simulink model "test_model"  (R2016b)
settings: Solver=VariableStepAuto  StartTime=0.0  StopTime=runtime  RelTol=1e-3
InitFcn:
  | clear mex
  | delete test_model_sfun.mexw64
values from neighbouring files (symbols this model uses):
  g = 9.81    [modelParameters.m]    (also in analyzeIMU_data.m = 9.8; getMomentOfInertia.m = 9.80665)
  height_controlled_o = (((Rm*If +      + (((omega0_o * 2 * Rm * Kv * Kq       * Kd + 1)^2) - 1)/(4* Rm*Kv^2*Kq      *Kd))/Vb)*(Pmax- Pmin)+Pmin)    [modelParameters.m]
  If = 0.511    [modelParameters.m]    (also in thrustDragConstantCalculations.m = [If0; If1; If2; If3]; Kd_error.m = I_0 * sign(rotor_speed_0) + I_1 * rotor_speed_0 + I_2 * roto)
  Jreq = 4.2012e-05    [modelParameters.m]
  Jxx = 0.0130    (= 0.013)    [modelParameters.m]
  Jyy = 0.0140    (= 0.014)    [modelParameters.m]
  Jzz = 0.0285    [modelParameters.m]
  Kd = 1.0317e-7    (= 1.0317e-07)    [modelParameters.m]    (also in calcDragConstant.m = ((A'*A)^-1)*A'*b; thrustDragConstantCalculations.m = calcDragConstant(data, Pmin, Pmax, Rm, Kv, Kq, If); Kd_error.m)
  Kq = 96.3422    [modelParameters.m]    (also in thrustDragConstantCalculations.m; Kd_error.m)
  Kt = 8.6519e-6    (= 8.6519e-06)    [modelParameters.m]    (also in calcThrustConstant.m = ((A'*A)^(-1))*(A'*T); thrustDragConstantCalculations.m = calcThrustConstant(data))
  Kv = 96.3422    [modelParameters.m]    (also in thrustDragConstantCalculations.m; Kd_error.m)
  m = 1.244    [modelParameters.m]
  omega0_o = (-1 + sqrt(1 - 4*Rm*Kv*Kq*Kd*( Kv*Rm*If - Kv*Vb_eff_0))) / (2*Rm*Kv*Kq*Kd)    [modelParameters.m]
  omega1_o = (-1 + sqrt(1 - 4*Rm*Kv*Kq*Kd*( Kv*Rm*If - Kv*Vb_eff_1))) / (2*Rm*Kv*Kq*Kd)    [modelParameters.m]
  omega2_o = (-1 + sqrt(1 - 4*Rm*Kv*Kq*Kd*( Kv*Rm*If - Kv*Vb_eff_2))) / (2*Rm*Kv*Kq*Kd)    [modelParameters.m]
  omega3_o = (-1 + sqrt(1 - 4*Rm*Kv*Kq*Kd*( Kv*Rm*If - Kv*Vb_eff_3))) / (2*Rm*Kv*Kq*Kd)    [modelParameters.m]
  pitch_o = pitch_value(1)    [modelParameters.m]
  pitchrate_o = pitchrate_value(1)    [modelParameters.m]
  Pmax = 2e5    (= 200000)    [modelParameters.m]    (also in thrustDragConstantCalculations.m; Kd_error.m)
  Pmin = 1e5    (= 100000)    [modelParameters.m]    (also in thrustDragConstantCalculations.m; Kd_error.m)
  rhx = 0.16    [modelParameters.m]
  rhy = 0.16    [modelParameters.m]
  rhz = 0.03    [modelParameters.m]
  Rm = 0.2308    [modelParameters.m]    (also in thrustDragConstantCalculations.m; Kd_error.m)
  roll_o = roll_value(1)    [modelParameters.m]
  rollrate_o = rollrate_value(1)    [modelParameters.m]
  Tc = 0.04    [modelParameters.m]
  Tq = 0.005    [modelParameters.m]
  Vb = 11.1    [modelParameters.m]    (also in calcDragConstant.m = [data.(6); data.(6); data.(6); data.(6)]; Kd_error.m = data.(6))
  x_controlled_o = 0    [modelParameters.m]
  x_o = x_position(1)    [modelParameters.m]
  x_vel_o = (x_position(2) - x_position(1)) / (time(2) - time(1))    [modelParameters.m]
  y_controlled_o = 0    [modelParameters.m]
  y_o = y_position(1)    [modelParameters.m]
  y_vel_o = (y_position(2) - y_position(1)) / (time(2) - time(1))    [modelParameters.m]
  yaw_controlled_o = 0    [modelParameters.m]
  yaw_o = yaw_value(1)    [modelParameters.m]
  yawrate_o = yawrate_value(1)    [modelParameters.m]
  z_o = z_position(1)    [modelParameters.m]
  z_vel_o = (z_position(2) - z_position(1)) / (time(2) - time(1))    [modelParameters.m]
undefined symbols (not defined in the file or in its folder): DiscIntNeverNeededParam
libraries: simulink x13, vrlib x2
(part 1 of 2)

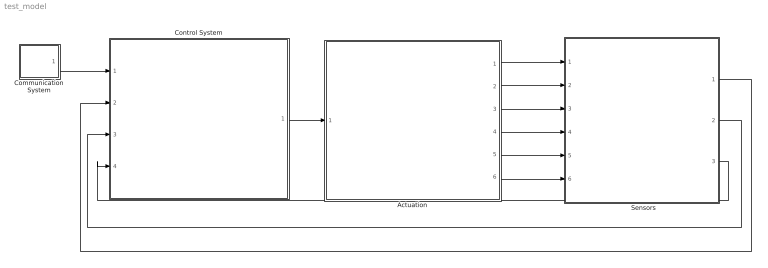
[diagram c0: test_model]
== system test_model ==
  "     Sensors   " : Subsystem
  Actuation : Subsystem
  Communication System : Subsystem
  Control System : Subsystem
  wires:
  Control System/1(P) -> Actuation/1(P)
  Communication System/1(setpoints) -> Control System/1(setpoints)
  Actuation/1(B_omega) -> "     Sensors   "/1(B_Omega)
  Actuation/2(euler_angles) -> "     Sensors   "/2(euler_angles)
  Actuation/3(B_vo) -> "     Sensors   "/3(B_vo)
  Actuation/4(E_ro) -> "     Sensors   "/4(E_ro)
  Actuation/5(B_vo_dot) -> "     Sensors   "/5(B_vo_dot)
  Actuation/6(B_g) -> "     Sensors   "/6(B_g)
  "     Sensors   "/3(current_position) -> Control System/4(current_position)
  "     Sensors   "/2(euler_rates) -> Control System/3(euler_rates)
  "     Sensors   "/1(euler_angles_filtered) -> Control System/2(euler_angles_filtered)

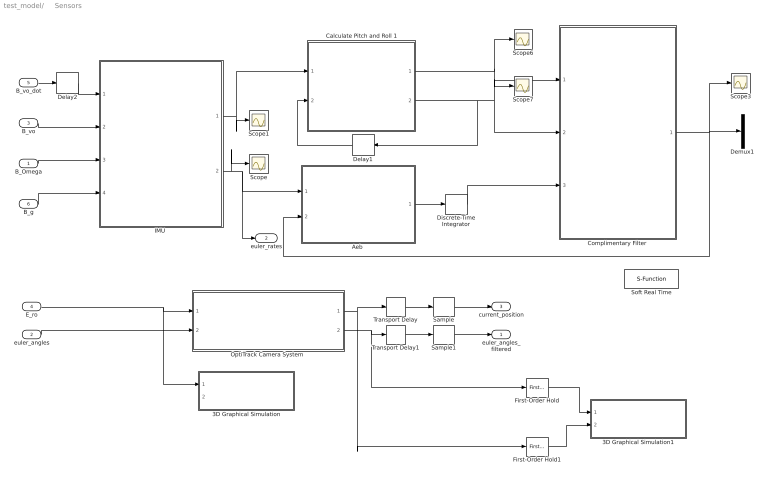
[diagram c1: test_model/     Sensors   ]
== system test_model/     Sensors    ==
  B_Omega : Inport
  euler_angles : Inport  Port=2
  B_vo : Inport  Port=3
  E_ro : Inport  Port=4
  B_vo_dot : Inport  Port=5
  B_g : Inport  Port=6
  3D Graphical Simulation : Subsystem  Commented=on
  3D Graphical Simulation1 : Subsystem  Commented=on
  "Aeb " : MATLAB Function  TreatAsAtomicUnit=on
  Calculate Pitch and Roll 1 : MATLAB Function  TreatAsAtomicUnit=on
  "Complimentary Filter " : MATLAB Function  TreatAsAtomicUnit=on
  Delay1 : Delay  DelayLength=1  InitialCondition=0  SampleTime=Tq
  Delay2 : Delay  DelayLength=1  InitialCondition=0  SampleTime=Tq
  Demux1 : Demux  Outputs=2
  Discrete-Time Integrator : DiscreteIntegrator  InitialConditionSetting=State (most efficient)  SampleTime=Tq  ICPrevOutput=DiscIntNeverNeededParam  ICPrevScaledInput=DiscIntNeverNeededParam
  First-Order Hold : simulink/Discrete/First-Order Hold  DisableCoverage=on  Ts=5e-3
  First-Order Hold1 : simulink/Discrete/First-Order Hold  DisableCoverage=on  Ts=5e-3
  "IMU " : Subsystem
  "OptiTrack Camera System " : Subsystem
  Sample : ZeroOrderHold  SampleTime=Tc
  Sample1 : ZeroOrderHold  SampleTime=Tc
  Scope{,1,3,6..7} (5 alike) : Scope
  Soft Real Time : S-Function  Commented=on  FunctionName=sfun_time  Parameters=x  SFunctionDeploymentMode=off  EnableBusSupport=off
  Transport Delay : TransportDelay  DelayTime=6e-3
  Transport Delay1 : TransportDelay  DelayTime=6e-3
  euler_angles_filtered : Outport
  euler_rates : Outport  Port=2
  current_position : Outport  Port=3
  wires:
  "IMU "/1(accelerometer) -> Calculate Pitch and Roll 1/1(accel_reading), Scope1/1
  "IMU "/2(gyroscope) -> Scope/1, euler_rates/1, "Aeb "/1(gyro_reading)
  B_vo/1 -> "IMU "/2(B_vo)
  B_Omega/1 -> "IMU "/3(B_Omega)
  B_g/1 -> "IMU "/4(B_g)
  Calculate Pitch and Roll 1/2(accel_roll) -> Scope7/1, "Complimentary Filter "/2(accel_roll), Delay1/1
  Calculate Pitch and Roll 1/1(accel_pitch) -> Scope6/1, "Complimentary Filter "/1(accel_pitch)
  Delay1/1 -> Calculate Pitch and Roll 1/2(accel_roll_prev)
  euler_angles/1 -> "OptiTrack Camera System "/2(yaw)
  First-Order Hold/1 -> 3D Graphical Simulation1/1("Euler Angles ")
  E_ro/1 -> 3D Graphical Simulation/1(Displacement), "OptiTrack Camera System "/1(E_ro)
  First-Order Hold1/1 -> 3D Graphical Simulation1/2(Displacement)
  B_vo_dot/1 -> Delay2/1
  Delay2/1 -> "IMU "/1(B_vo_dot)
  "Aeb "/1(euler_rates_IMU) -> Discrete-Time Integrator/1
  Discrete-Time Integrator/1 -> "Complimentary Filter "/3(euler_angles_gyro)
  "OptiTrack Camera System "/1(E_ro_camera) -> Transport Delay/1, First-Order Hold1/1
  "OptiTrack Camera System "/2(yaw_camera) -> First-Order Hold/1, Transport Delay1/1
  Transport Delay/1 -> Sample/1
  Transport Delay1/1 -> Sample1/1
  Sample/1 -> current_position/1
  Sample1/1 -> euler_angles_filtered/1
  "Complimentary Filter "/1(euler_angles_IMU) -> "Aeb "/2(euler_angles_IMU), Scope3/1, Demux1/1

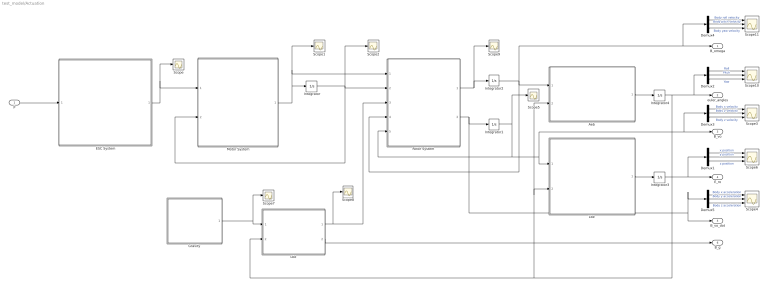
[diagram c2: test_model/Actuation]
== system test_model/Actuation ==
  P : Inport
  "Aeb " : MATLAB Function  TreatAsAtomicUnit=on
  Demux{1..5} (5 alike) : Demux  Outputs=3
  ESC System : MATLAB Function  TreatAsAtomicUnit=on
  "Gravity " : MATLAB Function  TreatAsAtomicUnit=on
  Integrator : Integrator  InitialCondition=[omega0_o, omega1_o, omega2_o, omega3_o]
  Integrator1 : Integrator  InitialCondition=[x_vel_o; y_vel_o; z_vel_o]
  Integrator2 : Integrator  InitialCondition=[rollrate_o; pitchrate_o; yawrate_o]
  Integrator3 : Integrator  InitialCondition=[x_o; y_o; z_o]
  Integrator4 : Integrator  InitialCondition=[roll_o; pitch_o; yaw_o]  ContinuousStateAttributes=['phi' 'theta' 'psi']
  "Lbe " : MATLAB Function  TreatAsAtomicUnit=on
  "Lbe " : MATLAB Function  TreatAsAtomicUnit=on
  Motor System : MATLAB Function  TreatAsAtomicUnit=on
  "Rotor System " : MATLAB Function  TreatAsAtomicUnit=on
  Scope{,1..2,5,7..9} (7 alike) : Scope
  Scope{3..4,6,10..11} (5 alike) : Scope  NumInputPorts=3
  B_omega : Outport
  euler_angles : Outport  Port=2
  B_vo : Outport  Port=3
  E_ro : Outport  Port=4
  B_vo_dot : Outport  Port=5
  B_g : Outport  Port=6
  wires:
  ESC System/1(Vb_eff) -> Scope/1, Motor System/1(Vb_eff)
  Motor System/1(w_dot) -> Integrator/1, "Rotor System "/1(w_dot), Scope1/1
  "Rotor System "/1(B_omega_dot) -> Scope9/1, Integrator2/1
  Integrator2/1 -> "Rotor System "/4(B_omega), B_omega/1, Demux4/1, "Aeb "/1(B_omega)
  "Aeb "/1(euler_rates) -> Integrator4/1
  "Lbe "/1(E_ro) -> Integrator3/1
  Integrator3/1 -> Demux1/1, E_ro/1
  "Lbe "/1(B_Fg) -> Scope8/1, "Rotor System "/3(B_Fg)
  "Lbe "/2(B_g) -> B_g/1
  Demux1/2 -> Scope6/2  "y position"
  Demux1/1 -> Scope6/1  "x position"
  Demux1/3 -> Scope6/3  "z position"
  Demux2/2 -> Scope10/2  "Pitch"
  Demux2/1 -> Scope10/1  "Roll"
  Demux2/3 -> Scope10/3  "Yaw"
  Demux4/2 -> Scope11/2  "Body pitch velocity"
  Demux4/1 -> Scope11/1  "Body roll velocity"
  Demux4/3 -> Scope11/3  "Body yaw velocity"
  Demux3/2 -> Scope3/2  "Body y velocity"
  Demux3/1 -> Scope3/1  "Body x velocity"
  Demux3/3 -> Scope3/3  "Body z velocity"
  Demux5/2 -> Scope4/2  "Body y acceleration"
  Demux5/1 -> Scope4/1  "Body x acceleration"
  Demux5/3 -> Scope4/3  "Body z acceleration"
  Integrator1/1 -> Scope5/1, "Rotor System "/5(B_vo), "Lbe "/1(B_vo), Demux3/1, B_vo/1
  "Rotor System "/2(B_vo_dot) -> Demux5/1, B_vo_dot/1, Integrator1/1
  Integrator4/1 -> euler_angles/1, Demux2/1, "Lbe "/2(euler_angles), "Aeb "/2(euler_angles), "Lbe "/2(euler_angles)
  P/1 -> ESC System/1(P)
  "Gravity "/1(E_Fg) -> Scope7/1, "Lbe "/1(E_Fg)
  Integrator/1 -> Motor System/2(w), "Rotor System "/2(w), Scope2/1

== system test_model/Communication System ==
  Step : Step  Before=[0; 0; 0; 0]  After=[1; 1; 0; 0]  SampleTime=Tq
  setpoints : Outport
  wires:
  Step/1 -> setpoints/1

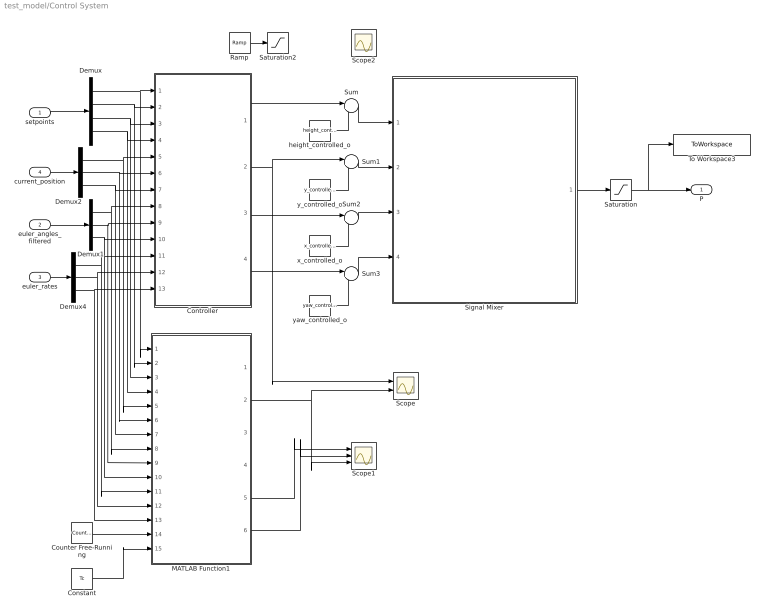
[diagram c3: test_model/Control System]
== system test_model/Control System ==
  setpoints : Inport
  euler_angles_filtered : Inport  Port=2
  euler_rates : Inport  Port=3
  current_position : Inport  Port=4
  Constant : Constant  Value=Tc  SampleTime=Tc
  Controller : Subsystem
  Counter Free-Running : simulink/Sources/Counter Free-Running  NumBits=32  tsamp=Tc
  Demux : Demux
  Demux1 : Demux  Outputs=3
  Demux2 : Demux  Outputs=3
  Demux4 : Demux  Outputs=3
  MATLAB Function1 : MATLAB Function  TreatAsAtomicUnit=on  SystemSampleTime=Tq
  Ramp : simulink/Sources/Ramp  slope=2*height_controlled_o  start=6.32  X0=0
  Saturation : Saturate  UpperLimit=Pmax*ones(4,1)  LowerLimit=Pmin*ones(4,1)
  Saturation2 : Saturate  UpperLimit=height_controlled_o  LowerLimit=0
  Scope : Scope  NumInputPorts=2
  Scope1 : Scope  NumInputPorts=3
  Scope2 : Scope
  Signal Mixer : MATLAB Function  TreatAsAtomicUnit=on
  Sum{,1..3} (4 alike) : Sum  Inputs=|++
  To Workspace3 : ToWorkspace  VariableName=motorCommands  SaveFormat=Structure With Time  SampleTime=Tq
  height_controlled_o : Constant  Value=height_controlled_o  SampleTime=Tc
  x_controlled_o : Constant  Value=x_controlled_o
  y_controlled_o : Constant  Value=y_controlled_o
  yaw_controlled_o : Constant  Value=yaw_controlled_o
  P : Outport
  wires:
  setpoints/1 -> Demux/1
  euler_angles_filtered/1 -> Demux1/1
  current_position/1 -> Demux2/1
  euler_rates/1 -> Demux4/1
  Demux/1 -> MATLAB Function1/1(set_x), Controller/1(x_setpoint)
  Demux/2 -> MATLAB Function1/2(set_y), Controller/2(y_setpoint)
  Demux/3 -> MATLAB Function1/3(set_z), Controller/3(z_setpoint)
  Demux2/1 -> MATLAB Function1/5(cur_x), Controller/5(x_position)
  Demux2/2 -> Controller/6(y_position), MATLAB Function1/6(cur_y)
  Demux2/3 -> MATLAB Function1/7(cur_z), Controller/7(z_position)
  Controller/2(y_controlled) -> Scope/1, Sum1/1
  Controller/4(yaw_controlled) -> Sum3/1
  y_controlled_o/1 -> Sum1/2
  x_controlled_o/1 -> Sum2/2
  yaw_controlled_o/1 -> Sum3/2
  Signal Mixer/1(P) -> Saturation/1
  Demux1/1 -> Controller/8(roll), MATLAB Function1/8(cur_phi)
  Demux1/2 -> MATLAB Function1/9(cur_theta), Controller/9(pitch)
  Demux4/1 -> Controller/11(roll_rate), MATLAB Function1/11(cur_phi_d)
  Demux4/2 -> Controller/12(pitch_rate), MATLAB Function1/12(cur_theta_d)
  Demux4/3 -> MATLAB Function1/13(cur_psi_d), Controller/13(yaw_rate)
  Demux/4 -> MATLAB Function1/4(set_yaw), Controller/4(yaw_setpoint)
  Demux1/3 -> MATLAB Function1/10(cur_psi), Controller/10(yaw)
  Controller/3(x_controlled) -> Sum2/1
  Counter Free-Running/1 -> MATLAB Function1/14(vrpn_id)
  Constant/1 -> MATLAB Function1/15(Tc)
  Sum/1 -> Signal Mixer/1(height_controlled)
  MATLAB Function1/5(pid_y_out) -> Scope1/1
  MATLAB Function1/6(pid_roll_out) -> Scope1/2
  MATLAB Function1/2(y_cor) -> Scope1/3, Scope/2
  Ramp/1 -> Saturation2/1
  height_controlled_o/1 -> Sum/2
  Saturation/1 -> To Workspace3/1, P/1
  Controller/1(height_controlled) -> Sum/1
  Sum1/1 -> Signal Mixer/2(y_controlled)
  Sum2/1 -> Signal Mixer/3(x_controlled)
  Sum3/1 -> Signal Mixer/4(yaw_controlled)

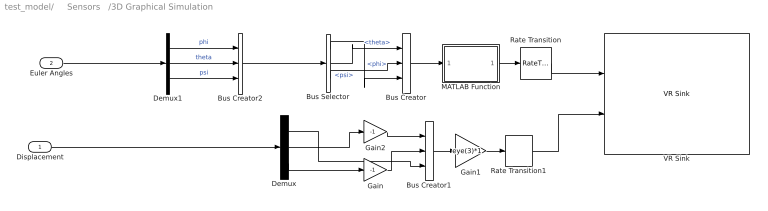
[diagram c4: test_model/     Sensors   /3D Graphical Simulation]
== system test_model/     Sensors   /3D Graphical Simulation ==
  Displacement : Inport
  Euler Angles : Inport  Port=2
  Bus Creator : BusCreator  Inputs=3
  Bus Creator1 : BusCreator  Inputs=3
  Bus Creator2 : BusCreator  Inputs=3
  Bus Selector : BusSelector  OutputSignals=phi,theta,psi
  Demux : Demux  Outputs=3
  Demux1 : Demux  Outputs=3
  Gain : Gain  Gain=-1
  Gain1 : Gain  Gain=eye(3)*1  Multiplication=Matrix(K*u)
  Gain2 : Gain  Gain=-1
  MATLAB Function : MATLAB Function  TreatAsAtomicUnit=on
  Rate Transition : RateTransition  OutPortSampleTime=0.06
  Rate Transition1 : RateTransition  OutPortSampleTime=0.06
  VR Sink : vrlib/VR Sink  InstantiateOnLoad=on  SampleTime=-1  ViewEnable=on  RemoteChange=off  RemoteView=off  FieldsWritten=Helicopter.rotation.4.1.1.double#Helicopter.translation.3.1.1.double  WorldFileName=quadrotor_world_ucart.wrl  AutoView=on  VideoDimensions=[]  AllowVariableSize=off
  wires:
  Displacement/1 -> Demux/1
  Bus Creator2/1 -> Bus Selector/1
  Demux/1 -> Bus Creator1/3
  Gain/1 -> Bus Creator1/2
  Gain2/1 -> Bus Creator1/1
  Rate Transition1/1 -> VR Sink/2
  Rate Transition/1 -> VR Sink/1
  Demux/3 -> Gain/1
  Demux/2 -> Gain2/1
  Bus Creator1/1 -> Gain1/1
  Bus Selector/1 -> Bus Creator/3  "<phi>"
  Bus Selector/3 -> Bus Creator/2  "<psi>"
  Bus Selector/2 -> Bus Creator/1  "<theta>"
  Gain1/1 -> Rate Transition1/1
  Demux1/3 -> Bus Creator2/3  "psi"
  Demux1/2 -> Bus Creator2/2  "theta"
  Demux1/1 -> Bus Creator2/1  "phi"
  Euler Angles/1 -> Demux1/1
  Bus Creator/1 -> MATLAB Function/1(u)
  MATLAB Function/1(y) -> Rate Transition/1

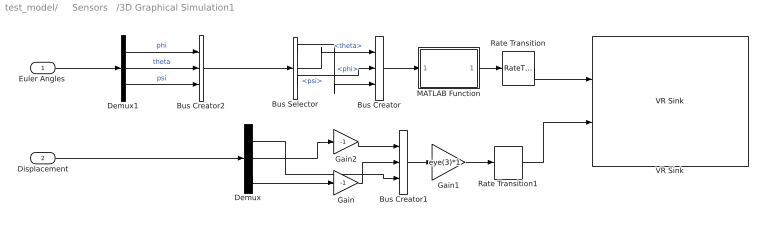
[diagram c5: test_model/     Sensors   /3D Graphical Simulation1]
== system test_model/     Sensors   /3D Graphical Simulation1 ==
  "Euler Angles " : Inport
  Displacement : Inport  Port=2
  Bus Creator : BusCreator  Inputs=3
  Bus Creator1 : BusCreator  Inputs=3
  Bus Creator2 : BusCreator  Inputs=3
  Bus Selector : BusSelector  OutputSignals=phi,theta,psi
  Demux : Demux  Outputs=3
  Demux1 : Demux  Outputs=3
  Gain : Gain  Gain=-1
  Gain1 : Gain  Gain=eye(3)*1  Multiplication=Matrix(K*u)
  Gain2 : Gain  Gain=-1
  MATLAB Function : MATLAB Function  TreatAsAtomicUnit=on
  Rate Transition : RateTransition  OutPortSampleTime=0.06
  Rate Transition1 : RateTransition  OutPortSampleTime=0.06
  VR Sink : vrlib/VR Sink  InstantiateOnLoad=on  SampleTime=-1  ViewEnable=on  RemoteChange=off  RemoteView=off  FieldsWritten=Helicopter.rotation.4.1.1.double#Helicopter.translation.3.1.1.double  WorldFileName=quadrotor_world_ucart.wrl  AutoView=on  VideoDimensions=[]  AllowVariableSize=off
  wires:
  Bus Creator2/1 -> Bus Selector/1
  Demux/1 -> Bus Creator1/3
  Gain/1 -> Bus Creator1/2
  Gain2/1 -> Bus Creator1/1
  Rate Transition1/1 -> VR Sink/2
  Rate Transition/1 -> VR Sink/1
  Demux/3 -> Gain/1
  Demux/2 -> Gain2/1
  Bus Creator1/1 -> Gain1/1
  Bus Selector/1 -> Bus Creator/3  "<phi>"
  Bus Selector/3 -> Bus Creator/2  "<psi>"
  Bus Selector/2 -> Bus Creator/1  "<theta>"
  Gain1/1 -> Rate Transition1/1
  Demux1/3 -> Bus Creator2/3  "psi"
  Demux1/2 -> Bus Creator2/2  "theta"
  Demux1/1 -> Bus Creator2/1  "phi"
  Bus Creator/1 -> MATLAB Function/1(u)
  MATLAB Function/1(y) -> Rate Transition/1
  Displacement/1 -> Demux/1
  "Euler Angles "/1 -> Demux1/1

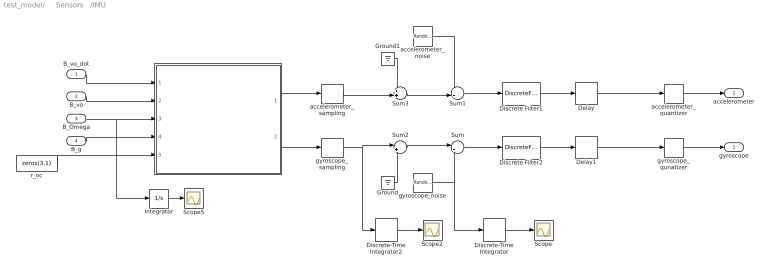
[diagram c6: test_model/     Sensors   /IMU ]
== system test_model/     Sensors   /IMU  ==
  B_vo_dot : Inport
  B_vo : Inport  Port=2
  B_Omega : Inport  Port=3
  B_g : Inport  Port=4
  " " : MATLAB Function  TreatAsAtomicUnit=on
  Delay : Delay  DelayLength=4  InitialCondition=0  SampleTime=Tq
  Delay1 : Delay  DelayLength=4  InitialCondition=0  SampleTime=Tq
  Discrete Filter1 : DiscreteFilter  Numerator=[0 0.1454]  Denominator=[1 -0.8546]  SampleTime=Tq
  Discrete Filter2 : DiscreteFilter  Numerator=[0 0.1454]  Denominator=[1 -0.8546]  SampleTime=Tq
  Discrete-Time Integrator : DiscreteIntegrator  InitialConditionSetting=State (most efficient)  SampleTime=-1  ICPrevOutput=DiscIntNeverNeededParam  ICPrevScaledInput=DiscIntNeverNeededParam
  Discrete-Time Integrator2 : DiscreteIntegrator  InitialConditionSetting=State (most efficient)  SampleTime=-1  ICPrevOutput=DiscIntNeverNeededParam  ICPrevScaledInput=DiscIntNeverNeededParam
  Ground : Ground
  Ground1 : Ground
  Integrator : Integrator
  Scope : Scope
  Scope2 : Scope
  Scope5 : Scope
  Sum : Sum  Inputs=|++
  Sum1 : Sum  Inputs=++|
  Sum2 : Sum  Inputs=|++
  Sum3 : Sum  Inputs=++|
  accelerometer_noise : RandomNumber  Mean=zeros(3,1)  Variance=[ 3e-7 ; 3.3e-7 ; 7.2e-7 ]  Seed=[0,1,2]  SampleTime=Tq
  accelerometer_quantizer : Quantizer  QuantizationInterval=2.4400e-04
  accelerometer_sampling : ZeroOrderHold  SampleTime=Tq
  gyroscope_noise : RandomNumber  Mean=zeros(3,1)  Variance=[ 2.2e-8 ; 1.1e-7 ; 2.4e-8 ]  Seed=[0,1,2]  SampleTime=Tq
  gyroscope_qunatizer : Quantizer  QuantizationInterval=1.1e-3
  gyroscope_sampling : ZeroOrderHold  SampleTime=Tq
  r_oc : Constant  Value=zeros(3,1)
  accelerometer : Outport
  gyroscope : Outport  Port=2
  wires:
  accelerometer_noise/1 -> Sum1/1
  Sum/1 -> Discrete Filter2/1
  Sum2/1 -> Sum/1
  Sum3/1 -> Sum1/2
  gyroscope_noise/1 -> Sum/2, Discrete-Time Integrator/1
  Sum1/1 -> Discrete Filter1/1
  gyroscope_sampling/1 -> Sum2/1, Discrete-Time Integrator2/1
  accelerometer_sampling/1 -> Sum3/2
  Ground/1 -> Sum2/2
  Ground1/1 -> Sum3/1
  B_vo_dot/1 -> " "/1(B_vo_dot)
  B_vo/1 -> " "/2(B_vo)
  B_Omega/1 -> Integrator/1, " "/3(B_Omega)
  B_g/1 -> " "/4(B_g)
  r_oc/1 -> " "/5(r_oc)
  " "/2(gyroReading) -> gyroscope_sampling/1
  " "/1(accelReading) -> accelerometer_sampling/1
  Discrete-Time Integrator/1 -> Scope/1
  Discrete-Time Integrator2/1 -> Scope2/1
  Integrator/1 -> Scope5/1
  gyroscope_qunatizer/1 -> gyroscope/1
  accelerometer_quantizer/1 -> accelerometer/1
  Discrete Filter2/1 -> Delay1/1
  Discrete Filter1/1 -> Delay/1
  Delay/1 -> accelerometer_quantizer/1
  Delay1/1 -> gyroscope_qunatizer/1

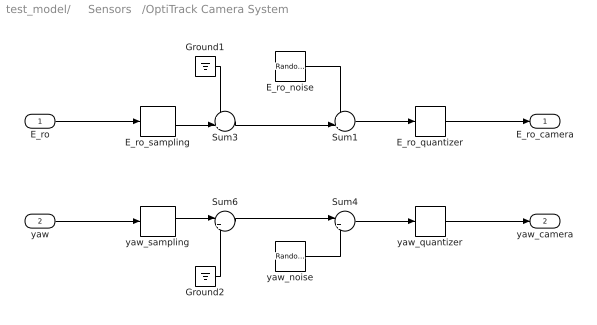
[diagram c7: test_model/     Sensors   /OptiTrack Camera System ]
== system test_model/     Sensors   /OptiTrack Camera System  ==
  E_ro : Inport
  yaw : Inport  Port=2
  E_ro_noise : RandomNumber  Mean=zeros(3,1)  Variance=[ 7.9664e-10 ; 1.1928e-10 ; 5.0636e-10 ]  Seed=[0,1,2]  SampleTime=Tc
  E_ro_quantizer : Quantizer  QuantizationInterval=2.4400e-04
  E_ro_sampling : ZeroOrderHold  SampleTime=Tc
  Ground1 : Ground
  Ground2 : Ground
  Sum1 : Sum  Inputs=++|
  Sum3 : Sum  Inputs=++|
  Sum4 : Sum  Inputs=|++
  Sum6 : Sum  Inputs=|++
  yaw_noise : RandomNumber  Variance=1.0783e-9  SampleTime=Tc
  yaw_quantizer : Quantizer  QuantizationInterval=1.1e-3
  yaw_sampling : ZeroOrderHold  SampleTime=Tc
  E_ro_camera : Outport
  yaw_camera : Outport  Port=2
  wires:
  E_ro_noise/1 -> Sum1/1
  Sum3/1 -> Sum1/2
  Sum1/1 -> E_ro_quantizer/1
  E_ro_sampling/1 -> Sum3/2
  Ground1/1 -> Sum3/1
  Sum4/1 -> yaw_quantizer/1
  Sum6/1 -> Sum4/1
  yaw_noise/1 -> Sum4/2
  yaw_sampling/1 -> Sum6/1
  Ground2/1 -> Sum6/2
  yaw/1 -> yaw_sampling/1
  E_ro/1 -> E_ro_sampling/1
  E_ro_quantizer/1 -> E_ro_camera/1
  yaw_quantizer/1 -> yaw_camera/1

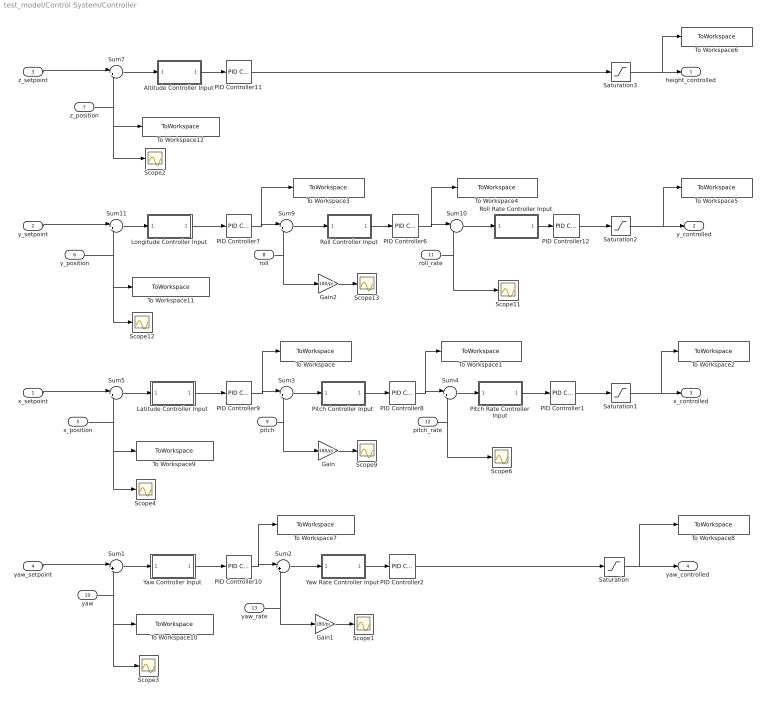
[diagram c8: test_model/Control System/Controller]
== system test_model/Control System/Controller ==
  x_setpoint : Inport
  y_setpoint : Inport  Port=2
  z_setpoint : Inport  Port=3
  yaw_setpoint : Inport  Port=4
  x_position : Inport  Port=5
  y_position : Inport  Port=6
  z_position : Inport  Port=7
  roll : Inport  Port=8
  pitch : Inport  Port=9
  yaw : Inport  Port=10
  roll_rate : Inport  Port=11
  pitch_rate : Inport  Port=12
  yaw_rate : Inport  Port=13
  Altitude Controller Input : Subsystem  Variant=on
  Gain : Gain  Gain=180/pi
  Gain1 : Gain  Gain=180/pi
  Gain2 : Gain  Gain=180/pi
  Latitude Controller Input : Subsystem  Variant=on
  Longitude Controller Input : Subsystem  Variant=on
  PID Controller1 : simulink/Continuous/PID Controller  Controller=P  TimeDomain=Discrete-time  SampleTime=Tq  IntegratorMethod=Forward Euler  FilterMethod=Forward Euler  Form=Parallel  UseFilter=off  ControllerParametersSource=internal  P=1835.12180866282  I=1575.82088970639  D=550  N=244.660686071579  InitialConditionSource=internal  InitialConditionForIntegrator=0  InitialConditionForFilter=0  ExternalReset=none  LimitOutput=off  UpperSaturationLimit=inf  LowerSaturationLimit=-inf  LinearizeAsGain=on  AntiWindupMode=none  Kb=1  TrackingMode=off  Kt=1  PParamMin=[]  PParamMax=[]  IParamMin=[]  IParamMax=[]  DParamMin=[]  DParamMax=[]  NParamMin=[]  NParamMax=[]  KbParamMin=[]  KbParamMax=[]  KtParamMin=[]  KtParamMax=[]  POutMin=[]  POutMax=[]  IOutMin=[]  IOutMax=[]  DOutMin=[]  DOutMax=[]  NOutMin=[]  NOutMax=[]  KbOutMin=[]  KbOutMax=[]  KtOutMin=[]  KtOutMax=[]  IntegratorOutMin=[]  IntegratorOutMax=[]  FilterOutMin=[]  FilterOutMax=[]  SumOutMin=[]  SumOutMax=[]  SumI1OutMin=[]  SumI1OutMax=[]  SumI2OutMin=[]  SumI2OutMax=[]  SumI3OutMin=[]  SumI3OutMax=[]  SumDOutMin=[]  SumDOutMax=[]  SaturationOutMin=[]  SaturationOutMax=[]  IntegratorContinuousStateAttributes=''  IntegratorStateMustResolveToSignalObject=off  IntegratorRTWStateStorageClass=Auto  FilterContinuousStateAttributes=''  FilterStateMustResolveToSignalObject=off  FilterRTWStateStorageClass=Auto  DifferentiatorICPrevScaledInput=0  DifferentiatorOutMin=[]  DifferentiatorOutMax=[]
  PID Controller10 : simulink/Continuous/PID Controller  Controller=PD  TimeDomain=Discrete-time  SampleTime=Tc  IntegratorMethod=Forward Euler  FilterMethod=Forward Euler  Form=Parallel  UseFilter=on  ControllerParametersSource=internal  P=4.73868196952772  I=2.36803176515497  D=1.0129554639517  N=3.83298618768959  InitialConditionSource=internal  InitialConditionForIntegrator=0  InitialConditionForFilter=0  ExternalReset=none  LimitOutput=off  UpperSaturationLimit=inf  LowerSaturationLimit=-inf  LinearizeAsGain=on  AntiWindupMode=none  Kb=1  TrackingMode=off  Kt=1  PParamMin=[]  PParamMax=[]  IParamMin=[]  IParamMax=[]  DParamMin=[]  DParamMax=[]  NParamMin=[]  NParamMax=[]  KbParamMin=[]  KbParamMax=[]  KtParamMin=[]  KtParamMax=[]  POutMin=[]  POutMax=[]  IOutMin=[]  IOutMax=[]  DOutMin=[]  DOutMax=[]  NOutMin=[]  NOutMax=[]  KbOutMin=[]  KbOutMax=[]  KtOutMin=[]  KtOutMax=[]  IntegratorOutMin=[]  IntegratorOutMax=[]  FilterOutMin=[]  FilterOutMax=[]  SumOutMin=[]  SumOutMax=[]  SumI1OutMin=[]  SumI1OutMax=[]  SumI2OutMin=[]  SumI2OutMax=[]  SumI3OutMin=[]  SumI3OutMax=[]  SumDOutMin=[]  SumDOutMax=[]  SaturationOutMin=[]  SaturationOutMax=[]  IntegratorContinuousStateAttributes=''  IntegratorStateMustResolveToSignalObject=off  IntegratorRTWStateStorageClass=Auto  FilterContinuousStateAttributes=''  FilterStateMustResolveToSignalObject=off  FilterRTWStateStorageClass=Auto  DifferentiatorICPrevScaledInput=0  DifferentiatorOutMin=[]  DifferentiatorOutMax=[]
  PID Controller11 : simulink/Continuous/PID Controller  Controller=PID  TimeDomain=Discrete-time  SampleTime=Tc  IntegratorMethod=Forward Euler  FilterMethod=Forward Euler  Form=Parallel  UseFilter=off  ControllerParametersSource=internal  P=-3138.91816077077  I=-320.189162634817  D=-7421.98260028101  N=5.79502261645411  InitialConditionSource=internal  InitialConditionForIntegrator=0  InitialConditionForFilter=0  ExternalReset=none  LimitOutput=off  UpperSaturationLimit=inf  LowerSaturationLimit=-inf  LinearizeAsGain=on  AntiWindupMode=none  Kb=1  TrackingMode=off  Kt=1  PParamMin=[]  PParamMax=[]  IParamMin=[]  IParamMax=[]  DParamMin=[]  DParamMax=[]  NParamMin=[]  NParamMax=[]  KbParamMin=[]  KbParamMax=[]  KtParamMin=[]  KtParamMax=[]  POutMin=[]  POutMax=[]  IOutMin=[]  IOutMax=[]  DOutMin=[]  DOutMax=[]  NOutMin=[]  NOutMax=[]  KbOutMin=[]  KbOutMax=[]  KtOutMin=[]  KtOutMax=[]  IntegratorOutMin=[]  IntegratorOutMax=[]  FilterOutMin=[]  FilterOutMax=[]  SumOutMin=[]  SumOutMax=[]  SumI1OutMin=[]  SumI1OutMax=[]  SumI2OutMin=[]  SumI2OutMax=[]  SumI3OutMin=[]  SumI3OutMax=[]  SumDOutMin=[]  SumDOutMax=[]  SaturationOutMin=[]  SaturationOutMax=[]  IntegratorContinuousStateAttributes=''  IntegratorStateMustResolveToSignalObject=off  IntegratorRTWStateStorageClass=Auto  FilterContinuousStateAttributes=''  FilterStateMustResolveToSignalObject=off  FilterRTWStateStorageClass=Auto  DifferentiatorICPrevScaledInput=0  DifferentiatorOutMin=[]  DifferentiatorOutMax=[]
  PID Controller12 : simulink/Continuous/PID Controller  Controller=P  TimeDomain=Discrete-time  SampleTime=Tq  IntegratorMethod=Forward Euler  FilterMethod=Forward Euler  Form=Parallel  UseFilter=off  ControllerParametersSource=internal  P=1835.12180866282  I=1575.82088970639  D=550  N=244.660686071579  InitialConditionSource=internal  InitialConditionForIntegrator=0  InitialConditionForFilter=0  ExternalReset=none  LimitOutput=off  UpperSaturationLimit=inf  LowerSaturationLimit=-inf  LinearizeAsGain=on  AntiWindupMode=none  Kb=1  TrackingMode=off  Kt=1  PParamMin=[]  PParamMax=[]  IParamMin=[]  IParamMax=[]  DParamMin=[]  DParamMax=[]  NParamMin=[]  NParamMax=[]  KbParamMin=[]  KbParamMax=[]  KtParamMin=[]  KtParamMax=[]  POutMin=[]  POutMax=[]  IOutMin=[]  IOutMax=[]  DOutMin=[]  DOutMax=[]  NOutMin=[]  NOutMax=[]  KbOutMin=[]  KbOutMax=[]  KtOutMin=[]  KtOutMax=[]  IntegratorOutMin=[]  IntegratorOutMax=[]  FilterOutMin=[]  FilterOutMax=[]  SumOutMin=[]  SumOutMax=[]  SumI1OutMin=[]  SumI1OutMax=[]  SumI2OutMin=[]  SumI2OutMax=[]  SumI3OutMin=[]  SumI3OutMax=[]  SumDOutMin=[]  SumDOutMax=[]  SaturationOutMin=[]  SaturationOutMax=[]  IntegratorContinuousStateAttributes=''  IntegratorStateMustResolveToSignalObject=off  IntegratorRTWStateStorageClass=Auto  FilterContinuousStateAttributes=''  FilterStateMustResolveToSignalObject=off  FilterRTWStateStorageClass=Auto  DifferentiatorICPrevScaledInput=0  DifferentiatorOutMin=[]  DifferentiatorOutMax=[]
  PID Controller2 : simulink/Continuous/PID Controller  Controller=P  TimeDomain=Discrete-time  SampleTime=Tc  IntegratorMethod=Forward Euler  FilterMethod=Forward Euler  Form=Parallel  UseFilter=on  ControllerParametersSource=internal  P=10205.7985086303  I=-77.7  D=2.32  N=1/0.0818  InitialConditionSource=internal  InitialConditionForIntegrator=0  InitialConditionForFilter=0  ExternalReset=none  ZeroCross=off  LimitOutput=off  UpperSaturationLimit=inf  LowerSaturationLimit=-inf  LinearizeAsGain=on  AntiWindupMode=none  Kb=1  TrackingMode=off  Kt=1  PParamMin=[]  PParamMax=[]  IParamMin=[]  IParamMax=[]  DParamMin=[]  DParamMax=[]  NParamMin=[]  NParamMax=[]  KbParamMin=[]  KbParamMax=[]  KtParamMin=[]  KtParamMax=[]  POutMin=[]  POutMax=[]  IOutMin=[]  IOutMax=[]  DOutMin=[]  DOutMax=[]  NOutMin=[]  NOutMax=[]  KbOutMin=[]  KbOutMax=[]  KtOutMin=[]  KtOutMax=[]  IntegratorOutMin=[]  IntegratorOutMax=[]  FilterOutMin=[]  FilterOutMax=[]  SumOutMin=[]  SumOutMax=[]  SumI1OutMin=[]  SumI1OutMax=[]  SumI2OutMin=[]  SumI2OutMax=[]  SumI3OutMin=[]  SumI3OutMax=[]  SumDOutMin=[]  SumDOutMax=[]  SaturationOutMin=[]  SaturationOutMax=[]  IntegratorContinuousStateAttributes=''  IntegratorStateMustResolveToSignalObject=off  IntegratorRTWStateStorageClass=Auto  FilterContinuousStateAttributes=''  FilterStateMustResolveToSignalObject=off  FilterRTWStateStorageClass=Auto  DifferentiatorICPrevScaledInput=0  DifferentiatorOutMin=[]  DifferentiatorOutMax=[]
  PID Controller6 : simulink/Continuous/PID Controller  Controller=P  TimeDomain=Discrete-time  SampleTime=Tc  IntegratorMethod=Forward Euler  FilterMethod=Forward Euler  Form=Parallel  UseFilter=off  ControllerParametersSource=internal  P=1  I=35.1207902652377  D=0.2  N=40.0107970227961  InitialConditionSource=internal  InitialConditionForIntegrator=0  InitialConditionForFilter=0  ExternalReset=none  LimitOutput=off  UpperSaturationLimit=inf  LowerSaturationLimit=-inf  LinearizeAsGain=on  AntiWindupMode=none  Kb=1  TrackingMode=off  Kt=1  PParamMin=[]  PParamMax=[]  IParamMin=[]  IParamMax=[]  DParamMin=[]  DParamMax=[]  NParamMin=[]  NParamMax=[]  KbParamMin=[]  KbParamMax=[]  KtParamMin=[]  KtParamMax=[]  POutMin=[]  POutMax=[]  IOutMin=[]  IOutMax=[]  DOutMin=[]  DOutMax=[]  NOutMin=[]  NOutMax=[]  KbOutMin=[]  KbOutMax=[]  KtOutMin=[]  KtOutMax=[]  IntegratorOutMin=[]  IntegratorOutMax=[]  FilterOutMin=[]  FilterOutMax=[]  SumOutMin=[]  SumOutMax=[]  SumI1OutMin=[]  SumI1OutMax=[]  SumI2OutMin=[]  SumI2OutMax=[]  SumI3OutMin=[]  SumI3OutMax=[]  SumDOutMin=[]  SumDOutMax=[]  SaturationOutMin=[]  SaturationOutMax=[]  IntegratorContinuousStateAttributes=''  IntegratorStateMustResolveToSignalObject=off  IntegratorRTWStateStorageClass=Auto  FilterContinuousStateAttributes=''  FilterStateMustResolveToSignalObject=off  FilterRTWStateStorageClass=Auto  DifferentiatorICPrevScaledInput=0  DifferentiatorOutMin=[]  DifferentiatorOutMax=[]
  PID Controller7 : simulink/Continuous/PID Controller  Controller=PD  TimeDomain=Discrete-time  SampleTime=Tc  IntegratorMethod=Forward Euler  FilterMethod=Forward Euler  Form=Parallel  UseFilter=on  ControllerParametersSource=internal  P=-0.00239291827793903  I=0.005  D=-0.101936697537801  N=33.9318377685715  InitialConditionSource=internal  InitialConditionForIntegrator=0  InitialConditionForFilter=0  ExternalReset=none  LimitOutput=off  UpperSaturationLimit=inf  LowerSaturationLimit=-inf  LinearizeAsGain=on  AntiWindupMode=none  Kb=1  TrackingMode=off  Kt=1  PParamMin=[]  PParamMax=[]  IParamMin=[]  IParamMax=[]  DParamMin=[]  DParamMax=[]  NParamMin=[]  NParamMax=[]  KbParamMin=[]  KbParamMax=[]  KtParamMin=[]  KtParamMax=[]  POutMin=[]  POutMax=[]  IOutMin=[]  IOutMax=[]  DOutMin=[]  DOutMax=[]  NOutMin=[]  NOutMax=[]  KbOutMin=[]  KbOutMax=[]  KtOutMin=[]  KtOutMax=[]  IntegratorOutMin=[]  IntegratorOutMax=[]  FilterOutMin=[]  FilterOutMax=[]  SumOutMin=[]  SumOutMax=[]  SumI1OutMin=[]  SumI1OutMax=[]  SumI2OutMin=[]  SumI2OutMax=[]  SumI3OutMin=[]  SumI3OutMax=[]  SumDOutMin=[]  SumDOutMax=[]  SaturationOutMin=[]  SaturationOutMax=[]  IntegratorContinuousStateAttributes=''  IntegratorStateMustResolveToSignalObject=off  IntegratorRTWStateStorageClass=Auto  FilterContinuousStateAttributes=''  FilterStateMustResolveToSignalObject=off  FilterRTWStateStorageClass=Auto  DifferentiatorICPrevScaledInput=0  DifferentiatorOutMin=[]  DifferentiatorOutMax=[]
  PID Controller8 : simulink/Continuous/PID Controller  Controller=P  TimeDomain=Discrete-time  SampleTime=Tc  IntegratorMethod=Forward Euler  FilterMethod=Forward Euler  Form=Parallel  UseFilter=off  ControllerParametersSource=internal  P=1  I=35.1207902652377  D=0.2  N=40.0107970227961  InitialConditionSource=internal  InitialConditionForIntegrator=0  InitialConditionForFilter=0  ExternalReset=none  LimitOutput=off  UpperSaturationLimit=inf  LowerSaturationLimit=-inf  LinearizeAsGain=on  AntiWindupMode=none  Kb=1  TrackingMode=off  Kt=1  PParamMin=[]  PParamMax=[]  IParamMin=[]  IParamMax=[]  DParamMin=[]  DParamMax=[]  NParamMin=[]  NParamMax=[]  KbParamMin=[]  KbParamMax=[]  KtParamMin=[]  KtParamMax=[]  POutMin=[]  POutMax=[]  IOutMin=[]  IOutMax=[]  DOutMin=[]  DOutMax=[]  NOutMin=[]  NOutMax=[]  KbOutMin=[]  KbOutMax=[]  KtOutMin=[]  KtOutMax=[]  IntegratorOutMin=[]  IntegratorOutMax=[]  FilterOutMin=[]  FilterOutMax=[]  SumOutMin=[]  SumOutMax=[]  SumI1OutMin=[]  SumI1OutMax=[]  SumI2OutMin=[]  SumI2OutMax=[]  SumI3OutMin=[]  SumI3OutMax=[]  SumDOutMin=[]  SumDOutMax=[]  SaturationOutMin=[]  SaturationOutMax=[]  IntegratorContinuousStateAttributes=''  IntegratorStateMustResolveToSignalObject=off  IntegratorRTWStateStorageClass=Auto  FilterContinuousStateAttributes=''  FilterStateMustResolveToSignalObject=off  FilterRTWStateStorageClass=Auto  DifferentiatorICPrevScaledInput=0  DifferentiatorOutMin=[]  DifferentiatorOutMax=[]
  PID Controller9 : simulink/Continuous/PID Controller  Controller=PD  TimeDomain=Discrete-time  SampleTime=Tc  IntegratorMethod=Forward Euler  FilterMethod=Forward Euler  Form=Parallel  UseFilter=on  ControllerParametersSource=internal  P=-0.00239291827793903  I=0.005  D=-0.101936697537801  N=33.9318377685715  InitialConditionSource=internal  InitialConditionForIntegrator=0  InitialConditionForFilter=0  ExternalReset=none  LimitOutput=off  UpperSaturationLimit=inf  LowerSaturationLimit=-inf  LinearizeAsGain=on  AntiWindupMode=none  Kb=1  TrackingMode=off  Kt=1  PParamMin=[]  PParamMax=[]  IParamMin=[]  IParamMax=[]  DParamMin=[]  DParamMax=[]  NParamMin=[]  NParamMax=[]  KbParamMin=[]  KbParamMax=[]  KtParamMin=[]  KtParamMax=[]  POutMin=[]  POutMax=[]  IOutMin=[]  IOutMax=[]  DOutMin=[]  DOutMax=[]  NOutMin=[]  NOutMax=[]  KbOutMin=[]  KbOutMax=[]  KtOutMin=[]  KtOutMax=[]  IntegratorOutMin=[]  IntegratorOutMax=[]  FilterOutMin=[]  FilterOutMax=[]  SumOutMin=[]  SumOutMax=[]  SumI1OutMin=[]  SumI1OutMax=[]  SumI2OutMin=[]  SumI2OutMax=[]  SumI3OutMin=[]  SumI3OutMax=[]  SumDOutMin=[]  SumDOutMax=[]  SaturationOutMin=[]  SaturationOutMax=[]  IntegratorContinuousStateAttributes=''  IntegratorStateMustResolveToSignalObject=off  IntegratorRTWStateStorageClass=Auto  FilterContinuousStateAttributes=''  FilterStateMustResolveToSignalObject=off  FilterRTWStateStorageClass=Auto  DifferentiatorICPrevScaledInput=0  DifferentiatorOutMin=[]  DifferentiatorOutMax=[]
  Pitch Controller Input : Subsystem  Variant=on
  Pitch Rate Controller Input : Subsystem  Variant=on
  Roll Controller Input : Subsystem  Variant=on
  Roll Rate Controller Input : Subsystem  Variant=on
  Saturation{,1..3} (4 alike) : Saturate  UpperLimit=30000  LowerLimit=-30000
  Scope{1..4,6,9,11..13} (9 alike) : Scope
  Sum{1..5,7,9..11} (9 alike) : Sum  Inputs=|+-
  To Workspace : ToWorkspace  VariableName=pitch_setpoint_model  SaveFormat=Structure With Time  SampleTime=-1
  To Workspace1 : ToWorkspace  VariableName=pitchrate_setpoint_model  SaveFormat=Structure With Time  SampleTime=-1
  To Workspace10 : ToWorkspace  VariableName=yaw_value_model  SaveFormat=Structure With Time  SampleTime=Tc
  To Workspace11 : ToWorkspace  VariableName=y_position_model  SaveFormat=Structure With Time  SampleTime=Tc
  To Workspace12 : ToWorkspace  VariableName=z_position_model  SaveFormat=Structure With Time  SampleTime=Tc
  To Workspace2 : ToWorkspace  VariableName=x_command_model  SaveFormat=Structure With Time  SampleTime=-1
  To Workspace3 : ToWorkspace  VariableName=roll_setpoint_model  SaveFormat=Structure With Time  SampleTime=Tc
  To Workspace4 : ToWorkspace  VariableName=rollrate_setpoint_model  SaveFormat=Structure With Time  SampleTime=Tc
  To Workspace5 : ToWorkspace  VariableName=y_command_model  SaveFormat=Structure With Time  SampleTime=Tq
  To Workspace6 : ToWorkspace  VariableName=z_command_model  SaveFormat=Structure With Time  SampleTime=Tc
  To Workspace7 : ToWorkspace  VariableName=yawrate_setpoint_model  SaveFormat=Structure With Time  SampleTime=Tc
  To Workspace8 : ToWorkspace  VariableName=yaw_command_model  SaveFormat=Structure With Time  SampleTime=Tc
  To Workspace9 : ToWorkspace  VariableName=x_position_model  SaveFormat=Structure With Time  SampleTime=Tc
  Yaw Controller Input : Subsystem  Variant=on
  Yaw Rate Controller Input : Subsystem  Variant=on
  height_controlled : Outport
  y_controlled : Outport  Port=2
  x_controlled : Outport  Port=3
  yaw_controlled : Outport  Port=4
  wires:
  pitch_rate/1 -> Scope6/1, Sum4/2
  z_setpoint/1 -> Sum7/1
  x_position/1 -> Scope4/1, To Workspace9/1, Sum5/2
  PID Controller8/1 -> Sum4/1, To Workspace1/1
  PID Controller9/1 -> Sum3/1, To Workspace/1
  pitch/1 -> Gain/1, Sum3/2
  Gain/1 -> Scope9/1
  PID Controller2/1 -> Saturation/1
  PID Controller1/1 -> Saturation1/1
  Latitude Controller Input/1(x_error) -> PID Controller9/1
  x_setpoint/1 -> Sum5/1
  roll_rate/1 -> Scope11/1, Sum10/2
  y_position/1 -> Scope12/1, To Workspace11/1, Sum11/2
  PID Controller6/1 -> Sum10/1, To Workspace4/1
  PID Controller7/1 -> Sum9/1, To Workspace3/1
  roll/1 -> Gain2/1, Sum9/2
  Gain2/1 -> Scope13/1
  PID Controller12/1 -> Saturation2/1
  y_setpoint/1 -> Sum11/1
  PID Controller11/1 -> Saturation3/1
  Saturation1/1 -> x_controlled/1, To Workspace2/1
  Saturation2/1 -> y_controlled/1, To Workspace5/1
  Saturation3/1 -> height_controlled/1, To Workspace6/1
  Saturation/1 -> yaw_controlled/1, To Workspace8/1
  yaw/1 -> Scope3/1, To Workspace10/1, Sum1/2
  yaw_setpoint/1 -> Sum1/1
  yaw_rate/1 -> Gain1/1, Sum2/2
  Gain1/1 -> Scope1/1
  PID Controller10/1 -> To Workspace7/1, Sum2/1
  z_position/1 -> To Workspace12/1, Scope2/1, Sum7/2
  Sum1/1 -> Yaw Controller Input/1(yaw_error_model)
  Yaw Controller Input/1(yaw_error) -> PID Controller10/1
  Sum2/1 -> Yaw Rate Controller Input/1(yawrate_error_model)
  Yaw Rate Controller Input/1(yawrate_error) -> PID Controller2/1
  Sum5/1 -> Latitude Controller Input/1(x_error_model)
  Sum3/1 -> Pitch Controller Input/1(pitch_error_model)
  Pitch Controller Input/1(pitch_error) -> PID Controller8/1
  Sum4/1 -> Pitch Rate Controller Input/1(pitchrate_error_model)
  Pitch Rate Controller Input/1(pitchrate_error) -> PID Controller1/1
  Sum11/1 -> Longitude Controller Input/1(y_error_model)
  Longitude Controller Input/1(y_error) -> PID Controller7/1
  Sum9/1 -> Roll Controller Input/1(roll_error_model)
  Roll Controller Input/1(roll_error) -> PID Controller6/1
  Sum10/1 -> Roll Rate Controller Input/1(rollrate_error_model)
  Roll Rate Controller Input/1(rollrate_error) -> PID Controller12/1
  Altitude Controller Input/1(z_error) -> PID Controller11/1
  Sum7/1 -> Altitude Controller Input/1(z_error_model)

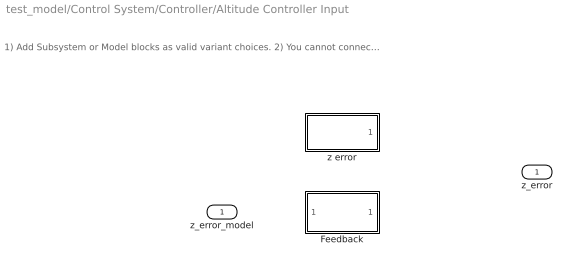
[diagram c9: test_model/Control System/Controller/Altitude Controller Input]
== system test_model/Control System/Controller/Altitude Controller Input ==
  note: 1) Add Subsystem or Model blocks as valid variant choices. 2) You cannot connect blocks at this level. At simulation, connectivity is automatically determined, based on the active variant and port name matching.
  z_error_model : Inport
  Feedback : Subsystem  VariantControl=logAnalysisToggle==0
  z error : Subsystem  VariantControl=logAnalysisToggle==1
  z_error : Outport

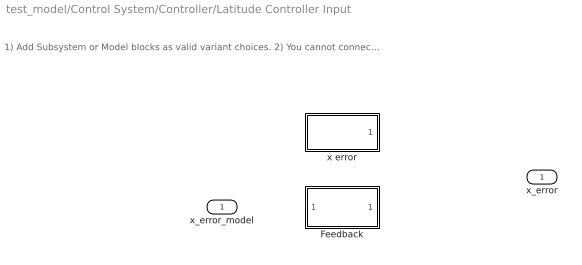
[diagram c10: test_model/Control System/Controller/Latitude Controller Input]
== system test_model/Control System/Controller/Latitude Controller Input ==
  note: 1) Add Subsystem or Model blocks as valid variant choices. 2) You cannot connect blocks at this level. At simulation, connectivity is automatically determined, based on the active variant and port name matching.
  x_error_model : Inport
  Feedback : Subsystem  VariantControl=logAnalysisToggle==0
  x error : Subsystem  VariantControl=logAnalysisToggle==1
  x_error : Outport

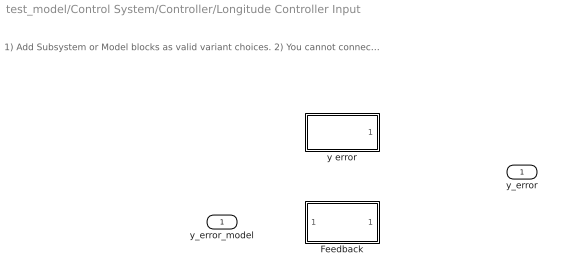
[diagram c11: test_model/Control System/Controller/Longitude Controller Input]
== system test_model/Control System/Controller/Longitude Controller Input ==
  note: 1) Add Subsystem or Model blocks as valid variant choices. 2) You cannot connect blocks at this level. At simulation, connectivity is automatically determined, based on the active variant and port name matching.
  y_error_model : Inport
  Feedback : Subsystem  VariantControl=logAnalysisToggle==0
  y error : Subsystem  VariantControl=logAnalysisToggle==1
  y_error : Outport

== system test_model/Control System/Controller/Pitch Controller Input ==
  note: 1) Add Subsystem or Model blocks as valid variant choices. 2) You cannot connect blocks at this level. At simulation, connectivity is automatically determined, based on the active variant and port name matching.
  pitch_error_model : Inport
  Feedback : Subsystem  VariantControl=logAnalysisToggle==0
  pitch error : Subsystem  VariantControl=logAnalysisToggle==1
  pitch_error : Outport

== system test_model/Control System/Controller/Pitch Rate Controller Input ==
  note: 1) Add Subsystem or Model blocks as valid variant choices. 2) You cannot connect blocks at this level. At simulation, connectivity is automatically determined, based on the active variant and port name matching.
  pitchrate_error_model : Inport
  Feedback : Subsystem  VariantControl=logAnalysisToggle==0
  pitchrate error : Subsystem  VariantControl=logAnalysisToggle==1
  pitchrate_error : Outport

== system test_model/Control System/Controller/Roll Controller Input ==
  note: 1) Add Subsystem or Model blocks as valid variant choices. 2) You cannot connect blocks at this level. At simulation, connectivity is automatically determined, based on the active variant and port name matching.
  roll_error_model : Inport
  Feedback : Subsystem  VariantControl=logAnalysisToggle==0
  roll error : Subsystem  VariantControl=logAnalysisToggle==1
  roll_error : Outport

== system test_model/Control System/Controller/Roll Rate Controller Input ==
  note: 1) Add Subsystem or Model blocks as valid variant choices. 2) You cannot connect blocks at this level. At simulation, connectivity is automatically determined, based on the active variant and port name matching.
  rollrate_error_model : Inport
  Feedback : Subsystem  VariantControl=logAnalysisToggle==0
  rollrate error : Subsystem  VariantControl=logAnalysisToggle==1
  rollrate_error : Outport

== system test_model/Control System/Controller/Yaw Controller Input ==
  note: 1) Add Subsystem or Model blocks as valid variant choices. 2) You cannot connect blocks at this level. At simulation, connectivity is automatically determined, based on the active variant and port name matching.
  yaw_error_model : Inport
  Feedback : Subsystem  VariantControl=logAnalysisToggle==0
  yaw error : Subsystem  VariantControl=logAnalysisToggle==1
  yaw_error : Outport

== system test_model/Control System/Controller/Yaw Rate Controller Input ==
  note: 1) Add Subsystem or Model blocks as valid variant choices. 2) You cannot connect blocks at this level. At simulation, connectivity is automatically determined, based on the active variant and port name matching.
  yawrate_error_model : Inport
  Feedback : Subsystem  VariantControl=logAnalysisToggle==0
  yawrate error : Subsystem  VariantControl=logAnalysisToggle==1
  yawrate_error : Outport

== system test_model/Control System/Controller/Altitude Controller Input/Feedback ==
  z_error_model : Inport
  z_error : Outport
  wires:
  z_error_model/1 -> z_error/1

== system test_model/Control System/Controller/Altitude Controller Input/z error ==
  From Workspace6 : FromWorkspace  VariableName=z_error  SampleTime=Tc
  z_error : Outport
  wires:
  From Workspace6/1 -> z_error/1

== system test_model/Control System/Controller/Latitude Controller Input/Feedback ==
  x_error_model : Inport
  x_error : Outport
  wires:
  x_error_model/1 -> x_error/1

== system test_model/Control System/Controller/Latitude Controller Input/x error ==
  From Workspace : FromWorkspace  VariableName=x_error  SampleTime=Tc
  x_error : Outport
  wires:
  From Workspace/1 -> x_error/1

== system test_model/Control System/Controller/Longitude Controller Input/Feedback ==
  y_error_model : Inport
  y_error : Outport
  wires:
  y_error_model/1 -> y_error/1

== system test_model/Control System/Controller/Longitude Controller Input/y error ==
  From Workspace3 : FromWorkspace  VariableName=y_error  SampleTime=Tc
  y_error : Outport
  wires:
  From Workspace3/1 -> y_error/1

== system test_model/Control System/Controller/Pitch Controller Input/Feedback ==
  pitch_error_model : Inport
  pitch_error : Outport
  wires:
  pitch_error_model/1 -> pitch_error/1

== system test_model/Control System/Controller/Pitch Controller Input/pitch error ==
  From Workspace : FromWorkspace  VariableName=pitch_error  SampleTime=Tc
  pitch_error : Outport
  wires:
  From Workspace/1 -> pitch_error/1

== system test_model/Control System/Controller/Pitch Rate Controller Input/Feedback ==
  pitchrate_error_model : Inport
  pitchrate_error : Outport
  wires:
  pitchrate_error_model/1 -> pitchrate_error/1

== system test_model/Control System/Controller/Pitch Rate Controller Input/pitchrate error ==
  From Workspace2 : FromWorkspace  VariableName=pitchrate_error  SampleTime=Tq
  pitchrate_error : Outport
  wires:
  From Workspace2/1 -> pitchrate_error/1

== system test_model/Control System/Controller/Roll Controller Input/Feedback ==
  roll_error_model : Inport
  roll_error : Outport
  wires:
  roll_error_model/1 -> roll_error/1

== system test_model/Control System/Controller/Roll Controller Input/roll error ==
  From Workspace4 : FromWorkspace  VariableName=roll_error  SampleTime=Tc
  roll_error : Outport
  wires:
  From Workspace4/1 -> roll_error/1

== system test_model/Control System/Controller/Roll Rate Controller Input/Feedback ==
  rollrate_error_model : Inport
  rollrate_error : Outport
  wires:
  rollrate_error_model/1 -> rollrate_error/1

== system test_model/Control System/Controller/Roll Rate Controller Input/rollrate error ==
  From Workspace5 : FromWorkspace  VariableName=rollrate_error  SampleTime=Tq
  rollrate_error : Outport
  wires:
  From Workspace5/1 -> rollrate_error/1

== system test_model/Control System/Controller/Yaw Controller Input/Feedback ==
  yaw_error_model : Inport
  yaw_error : Outport
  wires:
  yaw_error_model/1 -> yaw_error/1

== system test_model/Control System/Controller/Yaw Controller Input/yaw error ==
  From Workspace7 : FromWorkspace  VariableName=yaw_error  SampleTime=Tc
  yaw_error : Outport
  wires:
  From Workspace7/1 -> yaw_error/1

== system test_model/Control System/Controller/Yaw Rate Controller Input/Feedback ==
  yawrate_error_model : Inport
  yawrate_error : Outport
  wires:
  yawrate_error_model/1 -> yawrate_error/1

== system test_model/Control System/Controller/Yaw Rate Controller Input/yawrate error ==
  From Workspace8 : FromWorkspace  VariableName=yawrate_error  SampleTime=Tc
  yawrate_error : Outport
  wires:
  From Workspace8/1 -> yawrate_error/1

== matlab function test_model/Actuation/Gravity

 ==
function E_Fg = gravity(m, g)

E_Fg = [0; 0; m*g];

== matlab function test_model/Actuation/Lbe





 ==
function E_ro  = linear_body_earth_conversion(B_vo, euler_angles)

euler_rates = zeros(3,1);
E_ro = zeros(3,1);

phi = euler_angles(1);
theta = euler_angles(2);
psi = euler_angles(3);

Leb = [cos(theta)*cos(psi), sin(phi)*sin(theta)*cos(psi)-cos(phi)*sin(psi), cos(phi)*sin(theta)*cos(psi)+sin(phi)*sin(psi); ...
       cos(theta)*sin(psi), sin(phi)*sin(theta)*sin(psi)+cos(phi)*cos(psi), cos(phi)*sin(theta)*sin(psi)-sin(phi)*cos(psi); ...
           -sin(theta)    ,                sin(phi)*cos(theta)            ,                 cos(phi)*cos(theta)           ];

E_ro = Leb * B_vo;

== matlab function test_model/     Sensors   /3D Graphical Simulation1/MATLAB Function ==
function y = eigenaxis_ucart(u)


if abs(u(1))< 0.0001
    u(1) = 0.0001;
end

if abs(u(2))< 0.0001
    u(2) = 0.0001;
end

if abs(u(3))< 0.0001
    u(3) = 0.0001;
end

u = [ -u(1); -u(2); u(3) ];% [Pitch, Yaw, Roll] 

C11 = cos(u(2))*cos(u(3));
C12 = cos(u(2))*sin(u(3));
C13 = -sin(u(2));
C21 = sin(u(1))*sin(u(2))*cos(u(3))-cos(u(1))*sin(u(3));
C22 = sin(u(1))*sin(u(2))*sin(u(3))+cos(u(1))*cos(u(3));
C23 = sin(u(1))*cos(u(2));
C31 = cos(u(1))*sin(u(2))*cos(u(3))+sin(u(1))*sin(u(3));
C32 = cos(u(1))*sin(u(2))*sin(u(3))-sin(u(1))*cos(u(3));
C33 = cos(u(1))*cos(u(2));
    
theta = acos(0.5*(C11+C22+C33-1));

e = [C23-C32; C31-C13; C12-C21]/(2*sin(theta));
    
y = [e; theta];

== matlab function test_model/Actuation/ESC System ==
function Vb_eff   = ESC(P, Pmin, Pmax, Vb)

P1 = P(1);
P2 = P(2);
P3 = P(3);
P4 = P(4);

% Define u_Pi for each of the rotors, limiting it to be greater than 0
% u_P0 = (rotor_0_duty_cycle/100 - Pmin) / (Pmax - Pmin);
% u_P1 = (rotor_1_duty_cycle/100 - Pmin) / (Pmax - Pmin);
% u_P2 = (rotor_2_duty_cycle/100 - Pmin) / (Pmax - Pmin);
% u_P3 = (rotor_3_duty_cycle/100 - Pmin) / (Pmax - Pmin);
u_P0 = (P1 - Pmin) / (Pmax - Pmin);
u_P1 = (P2 - Pmin) / (Pmax - Pmin);
u_P2 = (P3 - Pmin) / (Pmax - Pmin);
u_P3 = (P4 - Pmin) / (Pmax - Pmin);


% Determine the effective battery voltage from each ESC
Vb_eff_0 = u_P0 * Vb;
Vb_eff_1 = u_P1 * Vb;
Vb_eff_2 = u_P2 * Vb;
Vb_eff_3 = u_P3 * Vb;
    
Vb_eff = [Vb_eff_0, Vb_eff_1, Vb_eff_2, Vb_eff_3];

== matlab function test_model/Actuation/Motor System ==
function w_dot = motor(Vb_eff, w, Rm, Kv, Kq, Kd, If, Jreq)

% Define each motors effective battery voltage
Vb_eff_0 = Vb_eff(1);
Vb_eff_1 = Vb_eff(2);
Vb_eff_2 = Vb_eff(3);
Vb_eff_3 = Vb_eff(4);

% Determine the angular velocity of each rotor from feedback
w_0 = w(1);
w_1 = w(2);
w_2 = w(3);
w_3 = w(4);

% Determine angular acceleration of each rotor
w_0_dot = 1/(Jreq*Rm*Kq) * Vb_eff_0 - 1/(Jreq*Rm*Kq*Kv) * w_0 - 1/(Jreq*Kq)*If - (Kd/Jreq) * w_0^2;
w_1_dot = 1/(Jreq*Rm*Kq) * Vb_eff_1 - 1/(Jreq*Rm*Kq*Kv) * w_1 - 1/(Jreq*Kq)*If - (Kd/Jreq) * w_1^2;
w_2_dot = 1/(Jreq*Rm*Kq) * Vb_eff_2 - 1/(Jreq*Rm*Kq*Kv) * w_2 - 1/(Jreq*Kq)*If - (Kd/Jreq) * w_2^2;
w_3_dot = 1/(Jreq*Rm*Kq) * Vb_eff_3 - 1/(Jreq*Rm*Kq*Kv) * w_3 - 1/(Jreq*Kq)*If - (Kd/Jreq) * w_3^2;

w_dot = [w_0_dot, w_1_dot, w_2_dot, w_3_dot];
